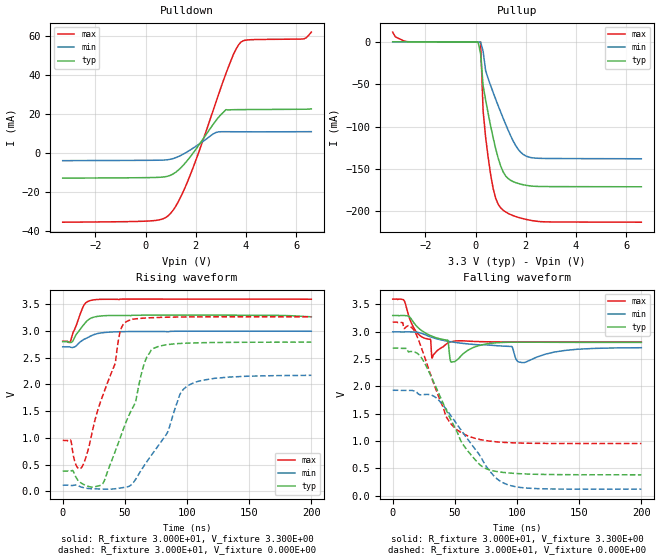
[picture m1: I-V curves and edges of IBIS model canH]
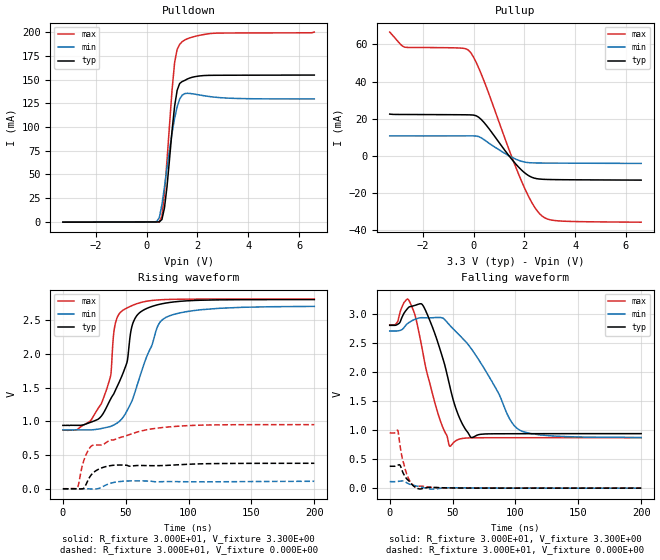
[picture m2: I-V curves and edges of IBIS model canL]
| IBIS file created by Layout Workbench Version 22.1.4.12161.401368   004
| Cadence Design Systems, Inc. 2011
[IBIS ver] 4.2
[File name]  tcan34xx.ibs
[File Rev]  1.0
[Date]   06 20, 2024
[Source] | Texas Instruments Incorporated.
[Notes] Revision History:
|   Component TCAN
[Component] TCAN
[Manufacturer] Manufacturer name
[Package]
| variable   typ   min   max
R_pkg   1.000E-01   8.000E-02   1.200E-01
L_pkg   1.000E-09   8.000E-10   1.200E-09
C_pkg   2.000E-13   1.600E-13   2.400E-13
[Pin]  signal_name   model_name   R_pin   L_pin   C_pin
Pin1   CANH   canH
Pin2   CANL   canL
Pin4   GND   Gnd
|Pin5  TXD_IN   dummy
Pin6   VCC   Power
|Pin6  EN   dummy
[Diff pin]  inv_pin  vdiff   tdelay_typ   tdelay_min   tdelay_max
CANL   CANH   2.200E+00  2.000E-08   1.500E-08   2.500E-08
| Models and submodels in the file (2): canH (Output), canL (Output)
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|   Model canH
[Model] canH
Model_type Output
Polarity   Inverting
Enable   Active-High
C_comp   4.254E-11   4.036E-11   4.819E-11
C_comp_pullup   1.635E-11   1.392E-11   1.694E-11
C_comp_pulldown   2.862E-11   2.401E-11   3.125E-11
[Temperature Range]   2.700E+01   1.500E+02   -5.500E+01
[Voltage Range]   3.300E+00   3.000E+00   3.600E+00
[Pullup Reference]   3.300E+00   3.000E+00   3.600E+00
[Pulldown Reference]   0.000E+00   0.000E+00   0.000E+00
[POWER Clamp Reference]   3.300E+00   3.000E+00   3.600E+00
[GND Clamp Reference]   0.000E+00   0.000E+00   0.000E+00
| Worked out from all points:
|   slope of the pulldown table from 0 to 0.495 V, typ, clamps not added: 3.35 kohm
|   slope of the pullup table from 0 to 0.495 V, typ, clamps not added: 5.92 ohm
|   rising waveform, R_fixture 3.000E+01, V_fixture 3.300E+00: 20-80 % time 9ns typ, 13.1ns min, 7.82ns max; typ from 2.8 V to 3.27 V
|   rising waveform, R_fixture 3.000E+01, V_fixture 0.000E+00: 20-80 % time 20.5ns typ, 26.6ns min, 17.8ns max; typ from 0.38 V to 2.79 V
|   falling waveform, R_fixture 3.000E+01, V_fixture 3.300E+00: 20-80 % time 17.3ns typ, 39.4ns min, 9.07ns max; typ from 3.29 V to 2.8 V
|   falling waveform, R_fixture 3.000E+01, V_fixture 0.000E+00: 20-80 % time 29.7ns typ, 33.6ns min, 21.6ns max; typ from 2.7 V to 0.381 V
[Pulldown]
|Voltage   I(typ)   I(min)   I(max)
-3.3V     -13mA      -4.009mA   -35.65mA
200mV     -12.71mA   -3.825mA   -34.99mA
900mV     -11.95mA   -3.498mA   -32.34mA
1.3V      -8.939mA   -1.938mA   -25.2mA
1.7V      -3.349mA   837.5uA    -13.91mA
2.7V      14.81mA    9.787mA    22.17mA
3V        19.66mA    10.87mA    33.58mA
3.2V      22.21mA    10.87mA    40.77mA
3.7V      22.23mA    10.85mA    55.52mA
4.1V      22.27mA    10.83mA    58.12mA
6.3V      22.43mA    10.88mA    58.62mA
6.6V      22.63mA    10.9mA     62.1mA
[Pullup]
|Voltage   I(typ)   I(min)   I(max)
-3.3V     378.5uA    319.7uA    11.85mA
-2.7V     325.2uA    281.3uA    424.9uA
100mV     144uA      135.7uA    116.3uA
200mV     -13.73mA   60.87uA    74.15uA
300mV     -51.52mA   -10.88mA   -81.47mA
400mV     -68.43mA   -33.64mA   -112.6mA
500mV     -84.28mA   -43.19mA   -136.3mA
800mV     -126.1mA   -67.59mA   -185mA
1.1V      -153.8mA   -90.24mA   -199.1mA
1.6V      -166.4mA   -122.6mA   -206.6mA
2.1V      -170mA     -135.9mA   -210.5mA
6.6V      -171.3mA   -138.1mA   -213.2mA
[Ramp]
| variable   typ   min   max
dV/dt_r   1.447E+00/2.047E-08   1.234E+00/2.658E-08   1.389E+00/1.776E-08
dV/dt_f   2.958E-01/1.733E-08   1.741E-01/3.941E-08   4.709E-01/9.050E-09
R_load = 3.000E+01
[Rising Waveform]
R_fixture= 3.000E+01
V_fixture= 3.300E+00
V_fixture_min= 3.000E+00
V_fixture_max= 3.600E+00
|time   V(typ)   V(min)   V(max)
0s        2.802V     2.705V     2.809V
4.68ns    2.793V     2.705V     2.789V
6.21ns    2.784V     2.698V     2.811V
8.04ns    2.809V     2.693V     2.949V
10.08ns   2.903V     2.708V     3.059V
16.92ns   3.12V      2.843V     3.477V
19.28ns   3.183V     2.868V     3.541V
24.17ns   3.254V     2.924V     3.581V
46.86ns   3.292V     2.988V     3.598V
200ns     3.267V     2.996V     3.595V
[Rising Waveform]
R_fixture= 3.000E+01
V_fixture= 0.000E+00
V_fixture_min= 0.000E+00
V_fixture_max= 0.000E+00
|time   V(typ)   V(min)   V(max)
0s        379.7mV    115mV      951.9mV
6.38ns    376.8mV    108.8mV    957.4mV
16.4ns    134.5mV    70.37mV    495.5mV
32.54ns   153.8mV    41.55mV    1.811V
42ns      734mV      47.2mV     2.379V
47ns      1.049V     64.78mV    3.048V
51.31ns   1.318V     79.55mV    3.178V
71.13ns   2.641V     668.8mV    3.249V
102.2ns   2.776V     1.997V     3.265V
200ns     2.792V     2.171V     3.266V
[Falling Waveform]
R_fixture= 3.000E+01
V_fixture= 3.300E+00
V_fixture_min= 3.000E+00
V_fixture_max= 3.600E+00
|time   V(typ)   V(min)   V(max)
0s        3.295V     2.996V     3.594V
8.65ns    3.296V     2.994V     3.583V
18.36ns   3.122V     2.991V     3.017V
30.4ns    2.927V     2.904V     2.859V
31.69ns   2.915V     2.894V     2.514V
44.32ns   2.842V     2.824V     2.791V
47.5ns    2.441V     2.812V     2.817V
95.77ns   2.806V     2.728V     2.811V
104.4ns   2.807V     2.434V     2.81V
200ns     2.802V     2.706V     2.809V
[Falling Waveform]
R_fixture= 3.000E+01
V_fixture= 0.000E+00
V_fixture_min= 0.000E+00
V_fixture_max= 0.000E+00
|time   V(typ)   V(min)   V(max)
0s        2.698V     1.927V     3.173V
15.68ns   2.637V     1.923V     3.065V
22.96ns   2.527V     1.844V     2.711V
33.01ns   2.076V     1.82V      2.048V
42.96ns   1.57V      1.582V     1.45V
57.99ns   888.8mV    1.106V     1.118V
73.03ns   517mV      618.1mV    1.014V
83.63ns   441.6mV    312.1mV    983.7mV
95.17ns   411.4mV    181.2mV    967.5mV
200ns     380.8mV    118.4mV    952.3mV
|   Model canL
[Model] canL
Model_type Output
Polarity   Non-Inverting
Enable   Active-High
C_comp   4.229E-11   4.062E-11   4.732E-11
C_comp_pullup   7.742E-13   5.739E-13   8.266E-13
C_comp_pulldown   4.172E-11   3.985E-11   4.649E-11
[Temperature Range]   2.700E+01   1.500E+02   -5.500E+01
[Voltage Range]   3.300E+00   3.000E+00   3.600E+00
[Pullup Reference]   3.300E+00   3.000E+00   3.600E+00
[Pulldown Reference]   0.000E+00   0.000E+00   0.000E+00
[POWER Clamp Reference]   3.300E+00   3.000E+00   3.600E+00
[GND Clamp Reference]   0.000E+00   0.000E+00   0.000E+00
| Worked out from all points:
|   slope of the pulldown table from 0 to 0.495 V, typ, clamps not added: 3.4 kohm
|   slope of the pullup table from 0 to 0.495 V, typ, clamps not added: 92.8 ohm
|   rising waveform, R_fixture 3.000E+01, V_fixture 3.300E+00: 20-80 % time 17.8ns typ, 20.7ns min, 11ns max; typ from 0.941 V to 2.8 V
|   rising waveform, R_fixture 3.000E+01, V_fixture 0.000E+00: 20-80 % time 11.2ns typ, 8.74ns min, 32ns max; typ from 0.003 V to 0.38 V
|   falling waveform, R_fixture 3.000E+01, V_fixture 3.300E+00: 20-80 % time 14.2ns typ, 27.4ns min, 13.2ns max; typ from 2.8 V to 0.941 V
|   falling waveform, R_fixture 3.000E+01, V_fixture 0.000E+00: 20-80 % time 7.32ns typ, 11.1ns min, 6.42ns max; typ from 0.38 V to 0.003 V
[Pulldown]
|Voltage   I(typ)   I(min)   I(max)
-3.3V     -266.7uA   -223uA     -316.6uA
300mV     -81.89uA   -26.1uA    -105.8uA
500mV     54.55uA    4.638mA    37.4uA
600mV     2.546mA    17.99mA    5.882mA
700mV     14.64mA    36.69mA    30.32mA
800mV     36.89mA    56.59mA    64.66mA
1V        96.3mA     93.71mA    139mA
1.1V      121.9mA    109.1mA    167.9mA
1.2V      138.7mA    121.3mA    181.7mA
1.4V      147.9mA    133.6mA    190mA
2.6V      154.5mA    131.6mA    198.7mA
6.6V      154.7mA    129.5mA    200mA
[Pullup]
|Voltage   I(typ)   I(min)   I(max)
-3.3V     22.5mA     10.78mA    66.62mA
-2.7V     22.3mA     10.77mA    58.47mA
-500mV    22.16mA    10.78mA    58.02mA
-100mV    22.07mA    10.8mA     55.38mA
100mV     21.63mA    10.72mA    50.43mA
400mV     18.2mA     8.892mA    40.76mA
1.4V      6.439uA    68.63uA    3.31mA
1.9V      -7.729mA   -2.919mA   -13.91mA
2.3V      -11.5mA    -3.716mA   -25.2mA
2.7V      -12.53mA   -3.815mA   -32.34mA
3.4V      -12.76mA   -3.867mA   -34.98mA
6.6V      -13mA      -4.023mA   -35.63mA
[Ramp]
| variable   typ   min   max
dV/dt_r   2.261E-01/1.118E-08   6.682E-02/8.741E-09   5.689E-01/3.204E-08
dV/dt_f   1.117E+00/1.420E-08   1.098E+00/2.740E-08   1.164E+00/1.318E-08
R_load = 3.000E+01
[Rising Waveform]
R_fixture= 3.000E+01
V_fixture= 3.300E+00
V_fixture_min= 3.000E+00
V_fixture_max= 3.600E+00
|time   V(typ)   V(min)   V(max)
0s        940.7mV    873.3mV    870.3mV
21.52ns   982.7mV    873.4mV    1V
30.48ns   1.075V     893.8mV    1.257V
38.05ns   1.332V     926.4mV    1.677V
41.91ns   1.464V     960.2mV    2.459V
49.87ns   1.812V     1.118V     2.666V
57.89ns   2.539V     1.463V     2.734V
75.38ns   2.725V     2.405V     2.796V
82.07ns   2.751V     2.54V      2.803V
200ns     2.802V     2.701V     2.809V
[Rising Waveform]
R_fixture= 3.000E+01
V_fixture= 0.000E+00
V_fixture_min= 0.000E+00
V_fixture_max= 0.000E+00
|time   V(typ)   V(min)   V(max)
0s        2.92mV     2.174mV    3.698mV
11.62ns   3.654mV    3.194mV    13.71mV
16.92ns   17.48mV    2.494mV    433.7mV
19.73ns   118.5mV    2.349mV    556.8mV
22.93ns   216.3mV    -24.78uV   638.1mV
31.27ns   314.4mV    30.32mV    653.5mV
36.92ns   342.1mV    77.98mV    716.9mV
63.01ns   347.3mV    119.2mV    861.2mV
105.5ns   369.6mV    106.2mV    941.9mV
200ns     379.8mV    113.5mV    951.8mV
[Falling Waveform]
R_fixture= 3.000E+01
V_fixture= 3.300E+00
V_fixture_min= 3.000E+00
V_fixture_max= 3.600E+00
|time   V(typ)   V(min)   V(max)
0s        2.802V     2.705V     2.809V
15.92ns   3.122V     2.859V     3.205V
20.24ns   3.147V     2.907V     2.969V
27.68ns   3.095V     2.933V     2.181V
38.06ns   2.521V     2.938V     1.309V
47.8ns    1.754V     2.803V     723.3mV
54.64ns   1.256V     2.65V      840.7mV
64.68ns   875.7mV    2.406V     868.3mV
103ns     939.2mV    1.006V     870.2mV
200ns     940.6mV    874.4mV    870.3mV
[Falling Waveform]
R_fixture= 3.000E+01
V_fixture= 0.000E+00
V_fixture_min= 0.000E+00
V_fixture_max= 0.000E+00
|time   V(typ)   V(min)   V(max)
0s        379.7mV    115mV      951.9mV
6.49ns    398.8mV    118.1mV    993.8mV
8.12ns    399.5mV    123.5mV    745.8mV
9.52ns    326.1mV    127.2mV    566.5mV
12.91ns   180.3mV    103.6mV    284mV
16.44ns   97.98mV    66.39mV    109.4mV
20.59ns   14.7mV     42.67mV    26.3mV
23.9ns    -10.84mV   30.18mV    36.68mV
33.28ns   16.2mV     -14.01mV   18.18mV
200ns     3.164mV    2.672mV    3.836mV
